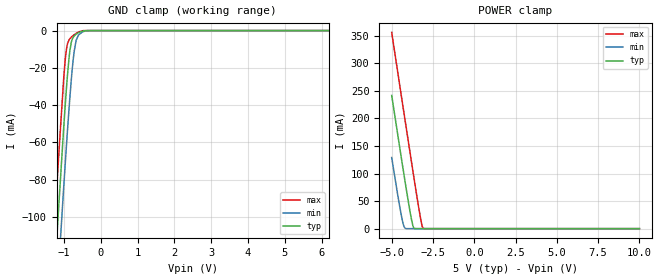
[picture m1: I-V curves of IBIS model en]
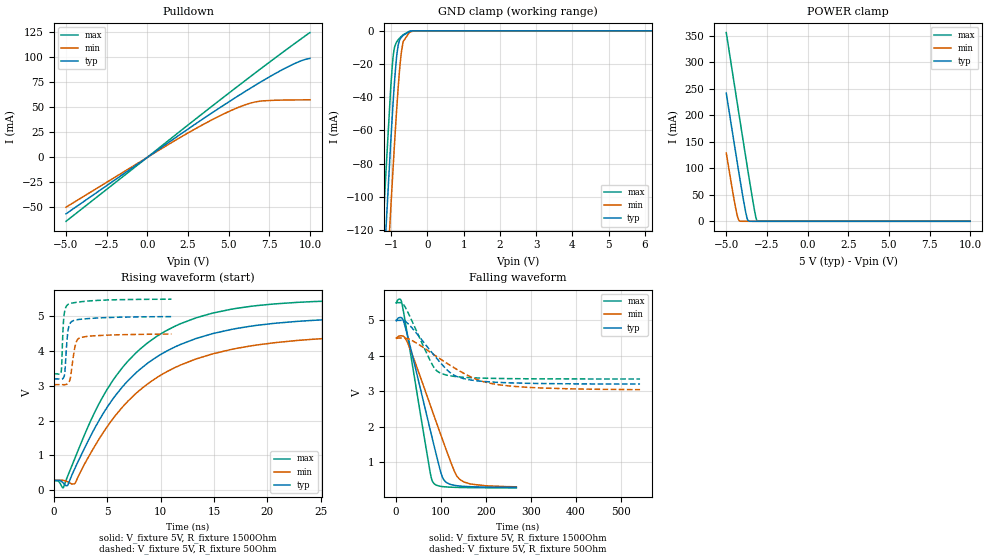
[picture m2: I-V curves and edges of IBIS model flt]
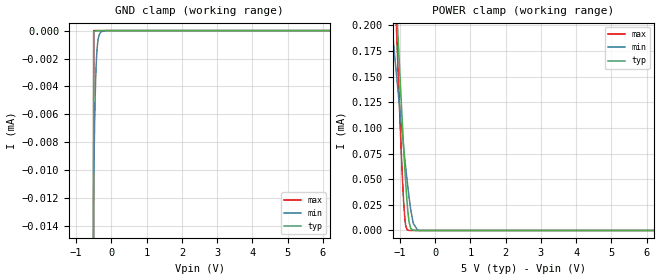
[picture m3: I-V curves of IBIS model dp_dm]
|Texas Instruments Incorporated
| AUTOMOTIVE USB 2.0 Interface Protection with Short-to-Battery and
| Short-to-Ground Protection
| Marketing part#   Digital Voltage Range   Package-type   #pins
| TPD3S714   4.5V-5.5V   DBQ   16
[IBIS Ver]   4.1
[File name]   tpd3s714.ibs
[File Rev]   1.0
[Date]   11/5/2015
[Source]
| Texas Instruments Incorporated.
| Analog-eLab Design Center, HPA
| 12500 TI Blvd
| Dallas, TX -75243
[Notes]   Revision History:
| Rev 1.0: 11/5/2015
| - Initial version of the model
| - Model generated from simulations in SPECTRE
| - Model matched to SPICE simulation
| - C_comp although listed in numerical order of value are
|   obtained from varying PVT conditions. For PVT conditions for
|   each specific value refer the buffer description under
|   respective [Model]. IBIS model user is responsible for using
|   appropriate C_comp to simulate for Signal Integrity.
[Disclaimer]
| This model is designed as an aid for customers of Texas Instruments.
| TI and its licensors and suppliers make no warranties, either expressed
| or implied, with respect to this  model, including the warranties of
| merchantability or fitness for a particular purpose. The model is
| provided solely on an "as is" basis. The entire risk as to its quality
| and performance is with the customer.
[Copyright]
(C) Copyright 2015 Texas Instruments Incorporated.All rights reserved.
|   TPD3S714
[Component]   TPD3S714
[Manufacturer]   TI
[Package]   |16 DBQ package
|   typ   min   max
R_pkg   0.1   0.08   0.12
L_pkg   1.0nH   0.8nH   1.2nH
C_pkg   0.2pF   0.16pF   0.24pF
[Pin]  signal_name   model_name   R_pin   L_pin   C_pin
1   NC   nc   na   na   na
2   Vbus_con   vbuscon   na   na   na
3   Vbus_con   vbuscon   na   na   na
4   GND   gnd   na   na   na
5   VD-   vdp_vdm   na   na   na
6   VD+   vdp_vdm   na   na   na
7   D-   dp_dm   na   na   na
8   D+   dp_dm   na   na   na
9   Vin   power   na   na   na
10   /FLT   flt   na   na   na
11   /EN   en   na   na   na
12   GND   gnd   na   na   na
13   GND   gnd   na   na   na
14   Vbus_sys   nc   na   na   na
15   Vbus_sys   nc   na   na   na
16   NC   nc   na   na   na
| Models and submodels in the file (5): en (Input), flt (I/O_open_drain), dp_dm (Terminator), vdp_vdm (Terminator), vbuscon (Terminator)
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|   en Model
[Model]   en
Model_type   Input
Vinl = 0.8
Vinh = 1.2
|   typ   min   max
|   (nom PVT)   (fast PVT)   (slow PVT)
C_comp   4.988e-13   4.811e-13   5.451e-13
| Where nom  PVT is Nominal Process, 5V, 40C
|   Fast PVT is Strong Process,  5.5V, -40C
|   Slow PVT is Weak Process,   4.5V, 125C
[Voltage Range]   5   4.5   5.5
|Junction Temperature
[Temperature Range]   40   125   -40
[Power Clamp Reference]   5   4.5   5.5
[GND Clamp Reference]   0   0   0
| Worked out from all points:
|   GND clamp passes 1 mA (typ) near -0.58 V on its own axis
|   POWER clamp passes 1 mA (typ) near -3.64 V on its own axis
[GND Clamp]
|   Voltage   I(typ)   I(min)   I(max)
-5V       -1.474A    -1.478A    -1.48A
-1.326V   -156.1mA   -187.5mA   -129.9mA
-1.247V   -129.6mA   -161.4mA   -102.7mA
-1.17V    -104.1mA   -136.3mA   -76.69mA
-1.145V   -95.98mA   -128.3mA   -68.43mA
-1.002V   -51.03mA   -83.05mA   -24.66mA
-919mV    -27.99mA   -58.41mA   -8.515mA
-836.5mV  -10.65mA   -35.69mA   -4.379mA
-750mV    -3.683mA   -16.07mA   -2.675mA
-666.5mV  -1.938mA   -5.201mA   -1.489mA
-603.5mV  -1.158mA   -2.357mA   -777uA
10V       0A         0A         0A
[POWER Clamp]
|   Voltage   I(typ)   I(min)   I(max)
-5V       241.8mA    129.1mA    356.3mA
-4.438V   132.6mA    27.27mA    245.3mA
-4.303V   106.8mA    8.374mA    218.8mA
-4.248V   96.5mA     3.521mA    208.2mA
-4.16V    79.82mA    420.1uA    190.8mA
-3.875V   28.4mA     142.5nA    135.2mA
-3.695V   3.579mA    32.19nA    100.4mA
-3.62V    400.4uA    31.36nA    86.03mA
-3.272V   0A         29.98nA    21.92mA
-3.163V   0A         29.62nA    5.604mA
-3.091V   0A         29.39nA    559.8uA
10V       0A         0A         0A
|   flt Model
[Model]   flt
Model_type   I/O_open_drain
Polarity   Non-Inverting
Vinl = 0.8
Vinh = 3.5
Vmeas = 2.5
Vref = 5
Cref = 2pF
Rref = 1500
|   typ   min   max
|   (nom PVT)   (fast PVT)   (slow PVT)
C_comp   5.357e-13   5.249e-13   5.856e-13
| Where nom  PVT is Nominal Process, 5V, 40C
|   Fast PVT is Strong Process,  5.5V, -40C
|   Slow PVT is Weak Process,   4.5V, 125C
[Voltage Range]   5   4.5   5.5
|Junction Temperature
[Temperature Range]   40   125   -40
[Pullup Reference]   5   4.5   5.5
[Pulldown Reference]   0   0   0
[Power Clamp Reference]   5   4.5   5.5
[GND Clamp Reference]   0   0   0
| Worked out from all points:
|   slope of the pulldown table from 0 to 0.75 V, typ, clamps not added: 86.9 ohm
|   GND clamp passes 1 mA (typ) near -0.54 V on its own axis
|   POWER clamp passes 1 mA (typ) near -3.64 V on its own axis
|   falling waveform, V_fixture 5V, R_fixture 1500Ohm: 20-80 % time 53.6ns typ, 70.8ns min, 40.7ns max; typ from 5 V to 0.282 V
|   rising waveform, V_fixture 5V, R_fixture 1500Ohm: 20-80 % time 8.01ns typ, 8.75ns min, 7.28ns max; typ from 0.275 V to 5 V
|   falling waveform, V_fixture 5V, R_fixture 50Ohm: 20-80 % time 71.8ns typ, 115ns min, 47.1ns max; typ from 5 V to 3.2 V
|   rising waveform, V_fixture 5V, R_fixture 50Ohm: 20-80 % time 283ps typ, 442ps min, 214ps max; typ from 3.2 V to 5 V
[Pulldown]
|   Voltage   I(typ)   I(min)   I(max)
-5V       -56.41mA   -49.77mA   -63.88mA
1.899V    21.62mA    18.77mA    24.64mA
3.744V    41.99mA    35.61mA    48.24mA
5.247V    58mA       47.59mA    67.2mA
6.322V    69.02mA    54.21mA    80.6mA
6.97V     75.41mA    56.31mA    88.59mA
8.935V    92.95mA    57.45mA    112.4mA
9.68V     97.83mA    57.55mA    121.1mA
10V       99.03mA    57.58mA    124.8mA
[GND Clamp]
|   Voltage   I(typ)   I(min)   I(max)
-5V       -1.862A    -1.873A    -1.865A
-1.225V   -152.8mA   -193.5mA   -118.4mA
-1.157V   -124.4mA   -165.4mA   -89.81mA
-1.012V   -66.87mA   -107.4mA   -34.04mA
-963mV    -48.7mA    -88.32mA   -19.23mA
-924.5mV  -35.64mA   -73.93mA   -11.78mA
-842mV    -13.8mA    -45.06mA   -6.434mA
-805mV    -8.404mA   -33.49mA   -5.324mA
-755mV    -5.02mA    -20.11mA   -4.096mA
-671mV    -2.758mA   -6.511mA   -2.391mA
-500mV    -522uA     -983.2uA   -256.6uA
10V       0A         0A         0A
[POWER Clamp]
|   Voltage   I(typ)   I(min)   I(max)
-5V       241.8mA    129.1mA    356.3mA
-4.438V   132.6mA    27.27mA    245.3mA
-4.303V   106.8mA    8.374mA    218.8mA
-4.248V   96.5mA     3.52mA     208.2mA
-4.16V    79.82mA    420.1uA    190.8mA
-3.875V   28.4mA     122.8nA    135.2mA
-3.695V   3.579mA    12.21nA    100.4mA
-3.62V    400.4uA    11.25nA    86.03mA
-3.272V   0A         0A         21.92mA
-3.163V   0A         0A         5.604mA
-3.091V   0A         0A         559.8uA
10V       0A         0A         0A
[Ramp]
R_load = 1500
|   typ   min   max
dV/dt_r   2.83519/8.00652e-09   2.53278/8.73001e-09   3.13904/7.28253e-09
dV/dt_f   2.8341/5.36473e-08   2.52913/7.09736e-08   3.13877/4.06087e-08
[Falling Waveform]
V_fixture = 5V
V_fixture_min = 4.5V
V_fixture_max = 5.5V
R_fixture = 1500Ohm
|   Time   V(typ)   V(min)   V(max)
0s        5V         4.5V       5.5V
8.488ns   5.083V     4.565V     5.602V
13.29ns   5.061V     4.564V     5.453V
32.33ns   4.217V     4.156V     4.043V
75.07ns   1.952V     2.641V     757.7mV
81.08ns   1.637V     2.425V     449.5mV
106.3ns   495.8mV    1.527V     302.2mV
130ns     341.3mV    732.2mV    285.5mV
141.4ns   322.5mV    512.7mV    281.7mV
267.6ns   281.6mV    299.7mV    270.4mV
[Rising Waveform]
V_fixture = 5V
V_fixture_min = 4.5V
V_fixture_max = 5.5V
R_fixture = 1500Ohm
|   Time   V(typ)   V(min)   V(max)
0s        274.7mV    278.6mV    268.3mV
877.2ps   202.9mV    276.8mV    59.15mV
1.266ns   122.9mV    237.4mV    373.2mV
1.935ns   595.7mV    177.2mV    881mV
4.411ns   2.094V     1.55V      2.586V
6.987ns   3.161V     2.571V     3.726V
10.45ns   3.98V      3.383V     4.576V
14.78ns   4.497V     3.913V     5.088V
27.14ns   4.928V     4.393V     5.457V
60.22ns   4.999V     4.498V     5.5V
[Falling Waveform]
V_fixture = 5V
V_fixture_min = 4.5V
V_fixture_max = 5.5V
R_fixture = 50Ohm
|   Time   V(typ)   V(min)   V(max)
0s        5V         4.5V       5.5V
16.26ns   4.997V     4.502V     5.453V
33.47ns   4.816V     4.444V     5.034V
79.29ns   4.098V     4.074V     3.778V
89.83ns   3.936V     3.983V     3.584V
102.5ns   3.75V      3.876V     3.492V
140.2ns   3.392V     3.58V      3.404V
179.7ns   3.295V     3.331V     3.375V
226.6ns   3.251V     3.187V     3.361V
543.2ns   3.202V     3.045V     3.346V
[Rising Waveform]
V_fixture = 5V
V_fixture_min = 4.5V
V_fixture_max = 5.5V
R_fixture = 50Ohm
|   Time   V(typ)   V(min)   V(max)
0s        3.2V       3.035V     3.345V
682.5ps   3.194V     3.035V     3.389V
720.7ps   3.195V     3.034V     3.502V
939.8ps   3.25V      3.032V     4.984V
1.029ns   3.38V      3.034V     5.17V
1.345ns   4.62V      3.078V     5.347V
1.569ns   4.822V     3.255V     5.376V
2.032ns   4.898V     4.191V     5.404V
2.453ns   4.917V     4.388V     5.422V
11.02ns   4.995V     4.493V     5.497V
|   dp_dm Model
[Model]   dp_dm
Model_type   Terminator
|   typ   min   max
|   (nom PVT)   (fast PVT)   (slow PVT)
C_comp   1.403e-12   1.401e-12   1.577e-12
| Where nom  PVT is Nominal Process, 5V, 40C
|   Fast PVT is Strong Process,  5.5V, -40C
|   Slow PVT is Weak Process,   4.5V, 125C
[Voltage Range]   5   4.5   5.5
|Junction Temperature
[Temperature Range]   40   125   -40
[Power Clamp Reference]   5   4.5   5.5
[GND Clamp Reference]   0   0   0
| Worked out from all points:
|   GND clamp passes 1 mA (typ) near -1.11 V on its own axis
[GND Clamp]
|   Voltage   I(typ)   I(min)   I(max)
-5V       -546.3mA   -432.3mA   -725.9mA
-1.101V   -911.5uA   -945.4uA   -1.68mA
-500mV    -97.47nA   -11.01uA   0A
-482mV    -61.46nA   -7.793uA   0A
-464mV    -40.04nA   -5.361uA   0A
-446mV    -27.01nA   -3.591uA   0A
-423.5mV  -17.14nA   -2.115uA   0A
-401mV    -11.14nA   -1.222uA   0A
-374mV    0A         -625.1nA   0A
-338mV    0A         -255.1nA   0A
-288.5mV  0A         -77.6nA    0A
10V       0A         0A         0A
[POWER Clamp]
|   Voltage   I(typ)   I(min)   I(max)
-5V       3.26mA     1.664mA    4.19mA
-1.235V   322.9uA    203.3uA    331.9uA
-1.105V   227.4uA    155.6uA    206.9uA
-1.073V   204.4uA    144.1uA    177uA
-990mV    145.9uA    114.5uA    102.4uA
-891.5mV  80.66uA    80.45uA    27.8uA
-830mV    44.72uA    60.17uA    4.269uA
-770.5mV  17.77uA    41.72uA    284.2nA
-690mV    2.004uA    20.06uA    5.85nA
-621.5mV  181.9nA    7.22uA     0A
-464mV    0A         141.2nA    0A
10V       0A         0A         0A
